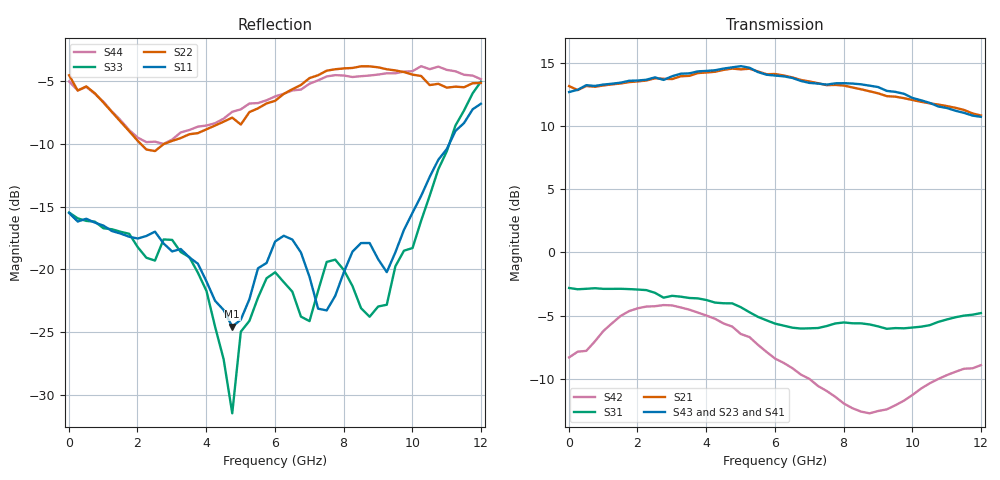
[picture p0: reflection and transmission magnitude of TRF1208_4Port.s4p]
! Created Thu Oct 27 02:43:40 2022
# hz S ri R 50
! 4 Port Network Data from SP1.SP block
! freq  reS11  imS11  reS12  imS12  reS13  imS13  reS14  imS14
!  reS21  imS21  reS22  imS22  reS23  imS23  reS24  imS24
!  reS31  imS31  reS32  imS32  reS33  imS33  reS34  imS34
!  reS41  imS41  reS42  imS42  reS43  imS43  reS44  imS44
!  Port-1 = INP
!  Port-3 = INM
!  Port-2 = OUTM
!  Port-4 = OUTP
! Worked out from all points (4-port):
!   49 points, 10 MHz to 12 GHz, reference 50 ohm
!   strongest paths, dB at 10 MHz, 3.01 GHz, 6.01 GHz, 9.01 GHz, 12 GHz:
!     S43: 12.7, 13.9, 14.0, 13.1, 10.7
!     S23: 13.0, 13.7, 13.9, 12.8, 10.5
!     S21: 13.1, 13.7, 14.1, 12.6, 10.8
!     S41: 12.9, 13.7, 14.0, 12.9, 11.0
!     S31: -2.8, -3.4, -5.6, -5.9, -4.8
!     S42: -8.3, -4.2, -8.4, -12.6, -8.9
!   lowest |S11| = -24.6 dB at 4.76 GHz (marker M1), VSWR 1.13, Z = 51.6 + j5.79 ohm
!   |S11| at or under -10 dB: start of sweep to 11.08 GHz
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1e7  -0.1622 -0.0429  0.0608 0.00288  0.6975 0.0236  0.0779 -0.00964
     4.533 0.3004  -0.5937 0.0199  -4.475 -0.1912  0.3747 0.0482
     0.7226 0.000914  0.0689 0.00214  -0.1685 0.00179  0.0632 0.000267
     -4.403 -0.2291  0.3833 -0.0246  4.306 0.0634  -0.5598 -0.0372
2.51e9  -0.1201 0.0746  0.0903 -0.0281  0.5764 -0.4285  0.1009 -0.0181
        3.648 -3.243  -0.2907 0.0565  -3.537 3.218  0.571 -0.2189
        0.5494 -0.4199  0.104 -0.0177  -0.0927 0.0561  0.0872 -0.0291
        -3.622 3.271  0.5699 -0.223  3.648 -3.304  -0.315 0.071
4.76e9  0.0191 0.0558  0.0678 -0.0817  0.1591 -0.6107  0.1047 -0.0672
        0.3347 -5.319  -0.3848 0.1183  -0.3879 5.24  0.2235 -0.4682
        0.1606 -0.6073  0.1093 -0.0669  0.00263 0.0265  0.0744 -0.079
        -0.3064 5.334  0.1954 -0.4694  0.3687 -5.379  -0.4107 0.1083
6.26e9  0.1346 0.0203  0.0238 -0.1152  -0.2241 -0.5056  0.074 -0.1146
        -2.458 -4.359  -0.4155 0.2793  2.267 4.399  -0.0738 -0.3768
        -0.1854 -0.4781  0.0778 -0.1171  0.088 -0.0123  0.0252 -0.1128
        2.583 4.196  -0.0691 -0.3586  -2.478 -4.305  -0.3883 0.3166
8.51e9  -0.0561 0.1143  -0.0767 -0.0649  -0.4944 0.0125  -0.018 -0.1071
        -4.306 -0.977  -0.1419 0.6289  4.317 1.232  -0.249 -0.0176
        -0.5226 0.0324  -0.0155 -0.1081  -0.0519 0.047  -0.0798 -0.0707
        4.408 1.058  -0.2333 -0.0225  -4.448 -1.244  -0.1055 0.5793
1.001e10  -0.1668 0.0216  -0.0781 -0.0186  -0.3829 0.3834  -0.0309 -0.0848
          -3.883 0.9751  -0.0926 0.5901  4.032 -0.9437  -0.1897 0.1812
          -0.3572 0.3556  -0.025 -0.0886  -0.1193 0.0236  -0.0768 -0.0182
          3.761 -1.168  -0.2112 0.1728  -3.89 1.227  -0.0473 0.6149
1.2e10  -0.4472 0.0946  -0.0414 0.0328  0.0779 0.5633  -0.0495 -0.067
        -1.486 3.144  -0.1153 0.5415  1.501 -3.009  -0.0274 0.3501
        0.0623 0.5715  -0.0516 -0.0624  -0.4961 0.2589  -0.0459 0.034
        1.511 -3.197  0.00471 0.3578  -1.463 3.108  -0.1475 0.5536
